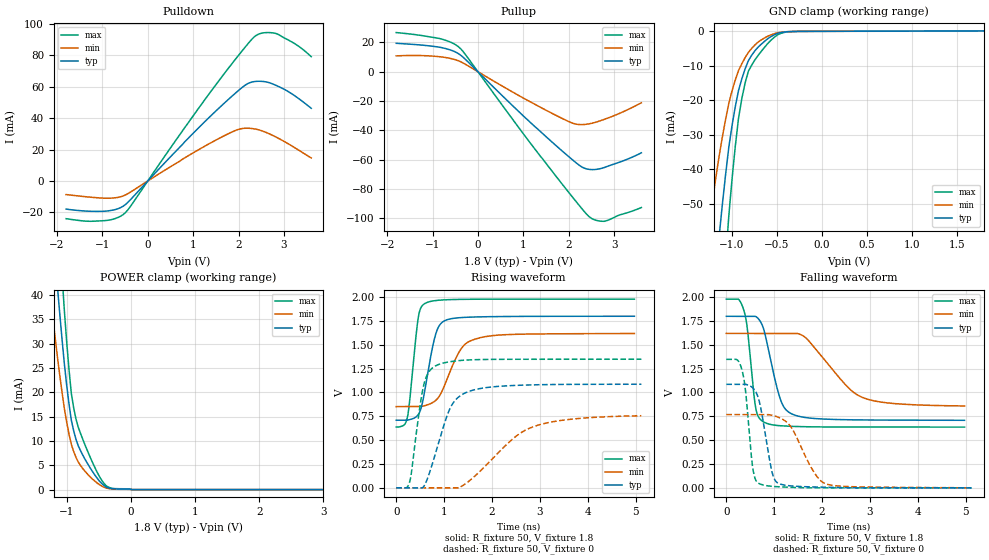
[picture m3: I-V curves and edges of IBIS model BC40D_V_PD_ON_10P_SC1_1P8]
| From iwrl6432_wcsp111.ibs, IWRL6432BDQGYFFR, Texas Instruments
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|   Model Cell BC40D_V_PD_ON_10P_SC1_1P8
|BC40D_V_PD_ON_10P_SC1_1P8
[Model]   BC40D_V_PD_ON_10P_SC1_1P8
Model_type   I/O
Polarity   Non-Inverting
Enable   Active-Low
Vinl =  0.63
Vinh =  1.17
Cref =  15pF
Rref =  100.0000M
Vref =  0V
Vmeas =  0.9
C_comp   2.290246p   2.205796p   2.292736p
|[Input load] weak_pd_on
|[Output drive] slow
|[supplytol] 10
|[temp] ind
[Model Spec]
Vinl   0.63   0.567   0.693
Vinh   1.17   1.053   1.287
[Temperature Range]   25   125   -40
[Voltage Range]   1.8   1.62   1.98
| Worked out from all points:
|   slope of the pulldown table from 0 to 0.27 V, typ, clamps not added: 32.2 ohm
|   slope of the pullup table from 0 to 0.27 V, typ, clamps not added: 32.6 ohm
|   GND clamp passes 1 mA (typ) near -0.53 V on its own axis
|   POWER clamp passes 1 mA (typ) near -0.43 V on its own axis
|   rising waveform, R_fixture 50, V_fixture 1.8: 20-80 % time 246ps typ, 417ps min, 160ps max; typ from 0.708 V to 1.8 V
|   rising waveform, R_fixture 50, V_fixture 0: 20-80 % time 429ps typ, 994ps min, 229ps max; typ from 0 V to 1.09 V
|   falling waveform, R_fixture 50, V_fixture 1.8: 20-80 % time 308ps typ, 788ps min, 165ps max; typ from 1.8 V to 0.708 V
|   falling waveform, R_fixture 50, V_fixture 0: 20-80 % time 226ps typ, 463ps min, 150ps max; typ from 1.08 V to 0 V
| Nom Voltages:
|   VDD=1.1001, VDDS=1.8, VDDS18=1.8, ESD_BIASFET=0, VSS=0, VSSS=0
| Min Voltages:
|   VDD=0.99, VDDS=1.62, VDDS18=1.62, ESD_BIASFET=0, VSS=0, VSSS=0
| Max Voltages:
|   VDD=1.21, VDDS=1.98, VDDS18=1.98, ESD_BIASFET=0, VSS=0, VSSS=0
[POWER_clamp]
|   voltage   I(typ)   I(min)   I(max)
-1.8V     158.9mA    112.6mA    219.9mA
-1.255V   60.04mA    40.04mA    85.04mA
-1.145V   41.99mA    27.45mA    59.9mA
-1.109V   36.4mA     23.66mA    51.96mA
-1.073V   31.03mA    20.08mA    44.3mA
-1.036V   25.91mA    16.71mA    36.9mA
-927.3mV  14.27mA    9.297mA    19.77mA
-854.5mV  10.33mA    6.619mA    14.49mA
-454.5mV  1.273mA    741.7uA    1.94mA
-309.1mV  221.6uA    132.8uA    307.9uA
18.18mV   0A         0A         0A
3.6V      0A         0A         0A
[Pulldown]
|   voltage   I(typ)   I(min)   I(max)
-1.8V     -17.92mA   -8.674mA   -24.03mA
-927.3mV  -19.22mA   -10.99mA   -25.2mA
-654.5mV  -17.65mA   -10.46mA   -23.22mA
-490.9mV  -14.97mA   -8.904mA   -20.12mA
818.2mV   25.05mA    14.78mA    34.16mA
1.691V    49.7mA     28.87mA    68.58mA
2.127V    60.63mA    33.53mA    84.59mA
2.4V      63.43mA    32.85mA    92.9mA
2.618V    62.99mA    30.74mA    94.47mA
2.836V    60.69mA    27.76mA    93.76mA
3.273V    53.49mA    20.53mA    86.73mA
3.6V      46.26mA    14.64mA    79.12mA
[Pullup]
|   voltage   I(typ)   I(min)   I(max)
-1.8V     19.42mA    10.82mA    26.76mA
-818.2mV  16.58mA    10.15mA    22.47mA
-545.5mV  14.19mA    8.648mA    19.37mA
-381.8mV  11.34mA    6.842mA    15.75mA
1.036V    -31.26mA   -18.6mA    -43.9mA
1.909V    -55.59mA   -32.73mA   -78.89mA
2.182V    -62.71mA   -35.92mA   -89.46mA
2.345V    -65.94mA   -36.05mA   -95.62mA
2.455V    -66.75mA   -35.58mA   -99.18mA
2.618V    -66.67mA   -34.29mA   -101.7mA
2.782V    -65.46mA   -32.56mA   -102.2mA
3.6V      -55.4mA    -21.22mA   -92.82mA
[GND_clamp]
|   voltage   I(typ)   I(min)   I(max)
-1.8V     -270.2mA   -170.2mA   -430.1mA
-1.255V   -91.66mA   -55.91mA   -148.4mA
-1.145V   -59.91mA   -36.45mA   -97.1mA
-1.109V   -50.48mA   -30.83mA   -81.56mA
-1.073V   -41.73mA   -25.65mA   -67.06mA
-1.036V   -33.67mA   -20.93mA   -53.6mA
-927.3mV  -17.08mA   -11.35mA   -25.06mA
-854.5mV  -10.88mA   -7.623mA   -14.95mA
-781.8mV  -6.944mA   -4.955mA   -9.81mA
-636.4mV  -2.852mA   -1.883mA   -4.568mA
-381.8mV  -107.5uA   -91.83uA   -158.4uA
1.8V      101.9uA    59.86uA    152.6uA
[Ramp]
| variable   typ   min   max
dV/dt_f 0.66096346/0.31032052n 0.46741953/0.81005029n 0.81000902/0.16620273n
dV/dt_r  0.6586759/0.43206812n 0.47399668/1.0503576n 0.81471515/0.23033778n
R_load = 50
[Rising Waveform]
R_fixture = 50
V_fixture = 1.8
V_fixture_min = 1.62
V_fixture_max = 1.98
|   time   V(typ)   V(min)   V(max)
0s        708.4mV    851.3mV    637.9mV
228.2ps   708.4mV    851.3mV    727.1mV
277.2ps   714.2mV    851.3mV    893.6mV
460ps     767.5mV    851.3mV    1.782V
607.4ps   1.051V     862.8mV    1.934V
832.2ps   1.622V     919.4mV    1.963V
1.059ns   1.761V     1.135V     1.971V
1.376ns   1.785V     1.471V     1.975V
1.754ns   1.792V     1.574V     1.977V
4.974ns   1.798V     1.617V     1.977V
[Rising Waveform]
R_fixture = 50
V_fixture = 0
V_fixture_min = 0
V_fixture_max = 0
|   time   V(typ)   V(min)   V(max)
0s        0V         0V         0V
277.1ps   0V         0V         55.7mV
567.1ps   9.209mV    0V         1.061V
665ps     114.2mV    0V         1.201V
831.9ps   380.6mV    0V         1.281V
1.154ns   861.6mV    0V         1.324V
1.542ns   1.015V     79.5mV     1.341V
2.435ns   1.072V     513.1mV    1.347V
2.83ns    1.079V     634.3mV    1.347V
5.119ns   1.086V     755.6mV    1.348V
[Falling Waveform]
R_fixture = 50
V_fixture = 1.8
V_fixture_min = 1.62
V_fixture_max = 1.98
|   time   V(typ)   V(min)   V(max)
0s        1.798V     1.619V     1.978V
367.8ps   1.798V     1.619V     1.858V
439.5ps   1.798V     1.619V     1.666V
613.8ps   1.796V     1.619V     836.4mV
784.1ps   1.656V     1.619V     689mV
1.123ns   936.1mV    1.619V     651.2mV
1.374ns   773.1mV    1.619V     644.4mV
1.662ns   736.2mV    1.571V     640.6mV
2.825ns   711.9mV    951.4mV    637.2mV
4.974ns   708.1mV    858.5mV    637mV
[Falling Waveform]
R_fixture = 50
V_fixture = 0
V_fixture_min = 0
V_fixture_max = 0
|   time   V(typ)   V(min)   V(max)
0s        1.085V     768.1mV    1.347V
222.8ps   1.085V     768.1mV    1.343V
331.6ps   1.085V     768.1mV    1.226V
405.7ps   1.085V     768.1mV    995.1mV
551.1ps   1.049V     768.1mV    212.2mV
682ps     917.5mV    768.1mV    45.69mV
951.1ps   172.2mV    761mV      16.04mV
1.106ns   43.25mV    735.9mV    11.02mV
2.086ns   5.683mV    40.73mV    0V
5.119ns   0V         0V         0V
